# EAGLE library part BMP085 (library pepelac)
BMP085 Digital pressure sensor
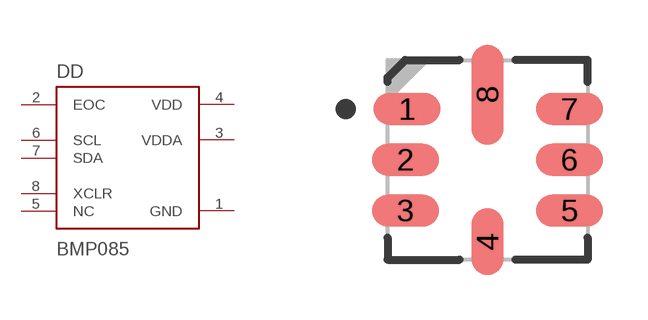
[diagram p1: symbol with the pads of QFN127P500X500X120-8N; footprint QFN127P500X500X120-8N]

Designator prefix DD

## BMP085  [QFN127P500X500X120-8N]
1  GND  pwr
2  EOC  out
3  VDDA  pwr
4  VDD  pwr
5  NC  nc
6  SCL  in
7  SDA
8  XCLR  in

## Footprint QFN127P500X500X120-8N (pad centres in mm)
IPC7351A / LCC8 / BMP085
smd 1.67 x 0.8: 1 -2.01,1.27; 2 -2.05,0; 3 -2.05,-1.27; 5 2.05,-1.27; 6 2.05,0; 7 2.05,1.27
smd 0.8 x 1.67: 4 0,-2.05
smd 0.8 x 2.5: 8 0,1.63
